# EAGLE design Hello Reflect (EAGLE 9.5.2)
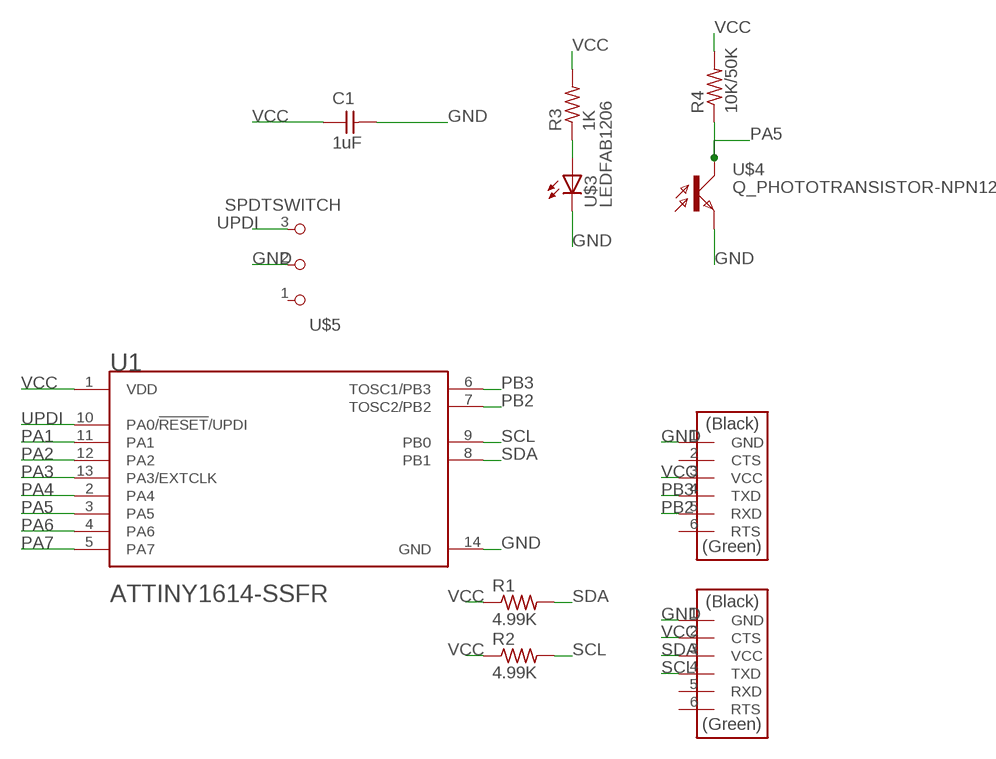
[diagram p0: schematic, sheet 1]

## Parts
C1  1uF  CAP_UNPOLARIZEDFAB  [C1206FAB]
R1  4.99K  R1206FAB  [R1206FAB]
R2  4.99K  R1206FAB  [R1206FAB]
R3  1K  R1206FAB  [R1206FAB]
R4  10K/50K  R1206FAB  [R1206FAB]
U1  MICROCHIP_ATTINY1614-SSFRMICROCHIP_ATTINY1614-SSFR_0_1  [MICROCHIP_ATTINY1614]
U$1  CONN_06_FTDI-SMD-HEADER  [1X06SMD]
U$2  CONN_06_FTDI-SMD-HEADER  [1X06SMD]
U$3  LEDFAB1206  [LED1206FAB]
U$4  Q_PHOTOTRANSISTOR-NPN1206  [OP1206]
U$5  SPDTSWITCH  [SPDTSWITCH]

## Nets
GND: C1.2 U1.14(GND) U$1.1(GND) U$2.1(GND) U$3.2(C) U$4.EMITTER(E) U$5.2
N$1: R3.1 U$3.1(A)
PA1: U1.11(PA1)
PA2: U1.12(PA2)
PA3: U1.13(PA3/EXTCLK)
PA4: U1.2(PA4)
PA5: R4.1 U1.3(PA5) U$4.COLLECTOR(C)
PA6: U1.4(PA6)
PA7: U1.5(PA7)
PB2: U1.7(TOSC2/PB2) U$2.5(RXD)
PB3: U1.6(TOSC1/PB3) U$2.4(TXD)
SCL: R2.2 U1.9(PB0) U$1.4(TXD)
SDA: R1.2 U1.8(PB1) U$1.3(VCC)
UPDI: U1.10(PA0/!RESET!/UPDI) U$5.3
VCC [New Class]: C1.1 R1.1 R2.1 R3.2 R4.2 U1.1(VDD) U$1.2(CTS) U$2.3(VCC)
Unconnected: U$1.5(RXD) U$1.6(RTS) U$2.2(CTS) U$2.6(RTS) U$5.1

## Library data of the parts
C1 = fab:CAP_UNPOLARIZED
R1-R4 = fab:R: Resistor (US Symbol)
U1 = Microchip - ATTINY1614-SSFR:MICROCHIP_ATTINY1614-SSFR: IC MCU 8BIT 16KB FLASH 14SOIC; AUTOMOTIVE: No; CENTROID_NOT_SPECIFIED: No; CORE_ARCHITECTURE: AVR; DATASHEET: http://ww1.microchip.com/downloads/en/DeviceDoc/ATtiny1614-DataSheet-DS40001995B.pdf; DATA_BUS_WIDTH: 8bits; DEVICE_CLASS_L1: Integrated Circuits (ICs); DEVICE_CLASS_L2: Embedded Processors and Controllers; DEVICE_CLASS_L3: Microcontrollers; DIGIKEY_DESCRIPTION: IC MCU 8BIT 16KB FLASH 14SOIC; DIGIKEY_PART_NUMBER: ATTINY1614-SSFRCT-ND; FOOTPRINT_PARAMETERS_1: {"fp_type":"SOIC_narrow","params":{"N":{"nom":14,"long name":"Number of leads","min":null,"max":null,"short name":"N","type":"count"},"A":{"nom":false,"long name":"Height","min":false,"max":1750000,"short name":"A","type":"measurement"},"A1":{"nom":false,"long name":"Package clearance","min":100000,"max":250000,"short name":"A1","type":"measurement"},"A2":{"nom":false,"long name":"Package height","min":1250000,"max":false,"short name":"A2","type":"measurement"},"D":{"nom":8650000,"long name":"Package length","min":8550000,"max":8750000,"short name":"D","type":"measurement"},"E":{"nom":6000000,"long name":"Width w/ leads","min":5800000,"max":6200000,"short name":"E","type":"measurement"},"E1":{"nom":3900000,"long name":"Package width","min":3800000,"max":4000000,"short name":"E1","type":"measurement"},"B":{"nom":false,"long name":"Lead width","min":310000,"max":510000,"short name":"B","type":"measurement"},"C":{"nom":false,"long name":"Lead thickness","min":100000,"max":250000,"short name":"C","type":"measurement"},"e":{"nom":1270000,"long name":"Lead pitch","min":null,"max":null,"short name":"e","type":"measurement"},"L":{"nom":false,"long name":"Lead foot length","min":400000,"max":1270000,"short name":"L","type":"measurement"},"PHI":{"nom":false,"long name":"Lead foot angle","min":0,"max":8000000,"short name":"PHI","type":"measurement"},"HT":{"default":"No","long name":"Thermal pad","type":"multichoiceparent","short name":"HT","children":[]},"offset x":{"nom":0,"long name":"X Center offset","min":null,"max":null,"short name":"offset x","type":"measurement"},"offset y":{"nom":0,"long name":"Y Center offset","min":null,"max":null,"short name":"offset y","type":"measurement"},"LS":{"default":"Rounded rectangle","long name":"Land shape","type":"multichoice","short name":"LS"},"LS1":{"default":"Rectangle","long name":"Land shape (Pin 1)","type":"multichoice","short name":"LS1"},"solder toe":{"nom":550000,"long name":"Solder fillet (toe)","min":null,"max":null,"short name":"solder toe","type":"fixedmeasurement"},"solder heel":{"nom":450000,"long name":"Solder fillet (heel)","min":null,"max":null,"short name":"solder heel","type":"fixedmeasurement"},"solder side":{"nom":50000,"long name":"Solder fillet (side)","min":null,"max":null,"short name":"solder side","type":"fixedmeasurement"},"courtyard":{"nom":500000,"long name":"Courtyard","min":null,"max":null,"short name":"courtyard","type":"fixedmeasurement"},"SF":{"default":"A","long name":"Packing level","type":"multichoiceparent","short name":"SF","help":"http://support.upverter.com/customer/portal/articles/978783-what-is-a-footprint-packing-level","children":["solder toe","solder heel","solder side","courtyard"]}}}; FOOTPRINT_PARAMETERS_2: {"fp_type":"SOIC_narrow","params":{"N":{"nom":14,"long name":"Number of leads","min":null,"max":null,"short name":"N","type":"count"},"A":{"nom":false,"long name":"Height","min":false,"max":1750000,"short name":"A","type":"measurement"},"A1":{"nom":false,"long name":"Package clearance","min":100000,"max":250000,"short name":"A1","type":"measurement"},"A2":{"nom":false,"long name":"Package height","min":1250000,"max":false,"short name":"A2","type":"measurement"},"D":{"nom":8650000,"long name":"Package length","min":8550000,"max":8750000,"short name":"D","type":"measurement"},"E":{"nom":6000000,"long name":"Width w/ leads","min":5800000,"max":6200000,"short name":"E","type":"measurement"},"E1":{"nom":3900000,"long name":"Package width","min":3800000,"max":4000000,"short name":"E1","type":"measurement"},"B":{"nom":false,"long name":"Lead width","min":310000,"max":510000,"short name":"B","type":"measurement"},"C":{"nom":false,"long name":"Lead thickness","min":100000,"max":250000,"short name":"C","type":"measurement"},"e":{"nom":1270000,"long name":"Lead pitch","min":null,"max":null,"short name":"e","type":"measurement"},"L":{"nom":false,"long name":"Lead foot length","min":400000,"max":1270000,"short name":"L","type":"measurement"},"PHI":{"nom":false,"long name":"Lead foot angle","min":0,"max":8000000,"short name":"PHI","type":"measurement"},"HT":{"default":"No","long name":"Thermal pad","type":"multichoiceparent","short name":"HT","children":[]},"offset x":{"nom":0,"long name":"X Center offset","min":null,"max":null,"short name":"offset x","type":"measurement"},"offset y":{"nom":0,"long name":"Y Center offset","min":null,"max":null,"short name":"offset y","type":"measurement"},"LS":{"default":"Rounded rectangle","long name":"Land shape","type":"multichoice","short name":"LS"},"LS1":{"default":"Rectangle","long name":"Land shape (Pin 1)","type":"multichoice","short name":"LS1"},"solder toe":{"nom":350000,"long name":"Solder fillet (toe)","min":null,"max":null,"short name":"solder toe","type":"fixedmeasurement"},"solder heel":{"nom":350000,"long name":"Solder fillet (heel)","min":null,"max":null,"short name":"solder heel","type":"fixedmeasurement"},"solder side":{"nom":30000,"long name":"Solder fillet (side)","min":null,"max":null,"short name":"solder side","type":"fixedmeasurement"},"courtyard":{"nom":250000,"long name":"Courtyard","min":null,"max":null,"short name":"courtyard","type":"fixedmeasurement"},"SF":{"default":"B","long name":"Packing level","type":"multichoiceparent","short name":"SF","help":"http://support.upverter.com/customer/portal/articles/978783-what-is-a-footprint-packing-level","children":["solder toe","solder heel","solder side","courtyard"]}}}; FOOTPRINT_PARAMETERS_3: {"fp_type":"SOIC_narrow","params":{"N":{"nom":14,"long name":"Number of leads","min":null,"max":null,"short name":"N","type":"count"},"A":{"nom":false,"long name":"Height","min":false,"max":1750000,"short name":"A","type":"measurement"},"A1":{"nom":false,"long name":"Package clearance","min":100000,"max":250000,"short name":"A1","type":"measurement"},"A2":{"nom":false,"long name":"Package height","min":1250000,"max":false,"short name":"A2","type":"measurement"},"D":{"nom":8650000,"long name":"Package length","min":8550000,"max":8750000,"short name":"D","type":"measurement"},"E":{"nom":6000000,"long name":"Width w/ leads","min":5800000,"max":6200000,"short name":"E","type":"measurement"},"E1":{"nom":3900000,"long name":"Package width","min":3800000,"max":4000000,"short name":"E1","type":"measurement"},"B":{"nom":false,"long name":"Lead width","min":310000,"max":510000,"short name":"B","type":"measurement"},"C":{"nom":false,"long name":"Lead thickness","min":100000,"max":250000,"short name":"C","type":"measurement"},"e":{"nom":1270000,"long name":"Lead pitch","min":null,"max":null,"short name":"e","type":"measurement"},"L":{"nom":false,"long name":"Lead foot length","min":400000,"max":1270000,"short name":"L","type":"measurement"},"PHI":{"nom":false,"long name":"Lead foot angle","min":0,"max":8000000,"short name":"PHI","type":"measurement"},"HT":{"default":"No","long name":"Thermal pad","type":"multichoiceparent","short name":"HT","children":[]},"offset x":{"nom":0,"long name":"X Center offset","min":null,"max":null,"short name":"offset x","type":"measurement"},"offset y":{"nom":0,"long name":"Y Center offset","min":null,"max":null,"short name":"offset y","type":"measurement"},"LS":{"default":"Rounded rectangle","long name":"Land shape","type":"multichoice","short name":"LS"},"LS1":{"default":"Rectangle","long name":"Land shape (Pin 1)","type":"multichoice","short name":"LS1"},"solder toe":{"nom":150000,"long name":"Solder fillet (toe)","min":null,"max":null,"short name":"solder toe","type":"fixedmeasurement"},"solder heel":{"nom":250000,"long name":"Solder fillet (heel)","min":null,"max":null,"short name":"solder heel","type":"fixedmeasurement"},"solder side":{"nom":10000,"long name":"Solder fillet (side)","min":null,"max":null,"short name":"solder side","type":"fixedmeasurement"},"courtyard":{"nom":100000,"long name":"Courtyard","min":null,"max":null,"short name":"courtyard","type":"fixedmeasurement"},"SF":{"default":"C","long name":"Packing level","type":"multichoiceparent","short name":"SF","help":"http://support.upverter.com/customer/portal/articles/978783-what-is-a-footprint-packing-level","children":["solder toe","solder heel","solder side","courtyard"]}}}; FOOTPRINT_VARIANT_NAME_0: Recommended_Land_Pattern; FOOTPRINT_VARIANT_NAME_1: IPC_A; FOOTPRINT_VARIANT_NAME_2: IPC_B; FOOTPRINT_VARIANT_NAME_3: IPC_C; FREQUENCY: 16MHz; HEIGHT: 1.75mm; INTERFACE: I2C,SPI,UART,USART,2-Wire,LIN,IrDA; IPC_LAND_PATTERN_NAME: SOIC127P600X175-14; LEAD_FREE: Yes; MAX_SUPPLY_VOLTAGE: 5.5V; MEMORY_SIZE: 16KBytes; MEMORY_TYPE: FLASH; MF: Microchip; MFG_PACKAGE_IDENT: C04-065-D3X; MFG_PACKAGE_IDENT_DATE: 0; MFG_PACKAGE_IDENT_REV: D; MIN_SUPPLY_VOLTAGE: 1.8V; MOUSER_DESCRIPTION: 8-Bit AVR Microcontroller 16Kbyte Flash 2Kbyte SRAM 14-Pin SOIC T/R; MOUSER_PART_NUMBER: 556-ATTINY1614SSFR; MPN: ATTINY1614-SSFR; NOMINAL_SUPPLY_CURRENT: 2.6-10200uA; NUMBER_OF_A/D_CONVERTERS: 2; NUMBER_OF_ADC_CHANNELS: 14; NUMBER_OF_CORES: 1; NUMBER_OF_I/OS: 12; NUMBER_OF_I2C_CHANNELS: 1; NUMBER_OF_PWM_CHANNELS: 1; NUMBER_OF_SPI_CHANNELS: 1; NUMBER_OF_TIMERS/COUNTERS: 5; NUMBER_OF_UART_CHANNELS: 1; PACKAGE: SOIC14; PREFIX: U; RAM_SIZE: 2KBytes; ROHS: Yes; STANDOFF_HEIGHT: 0.1mm; TEMPERATURE_RANGE_HIGH: +125°C; TEMPERATURE_RANGE_LOW: -40°C; VERIFICATION_VERSION: 0.0.0.3
U$1 U$2 = fab:CONN_06_FTDI-SMD-HEADER
U$3 = fab:LED: LED
U$4 = fab:Q_PHOTOTRANSISTOR-NPN
U$5 = fab:SPDTSWITCH

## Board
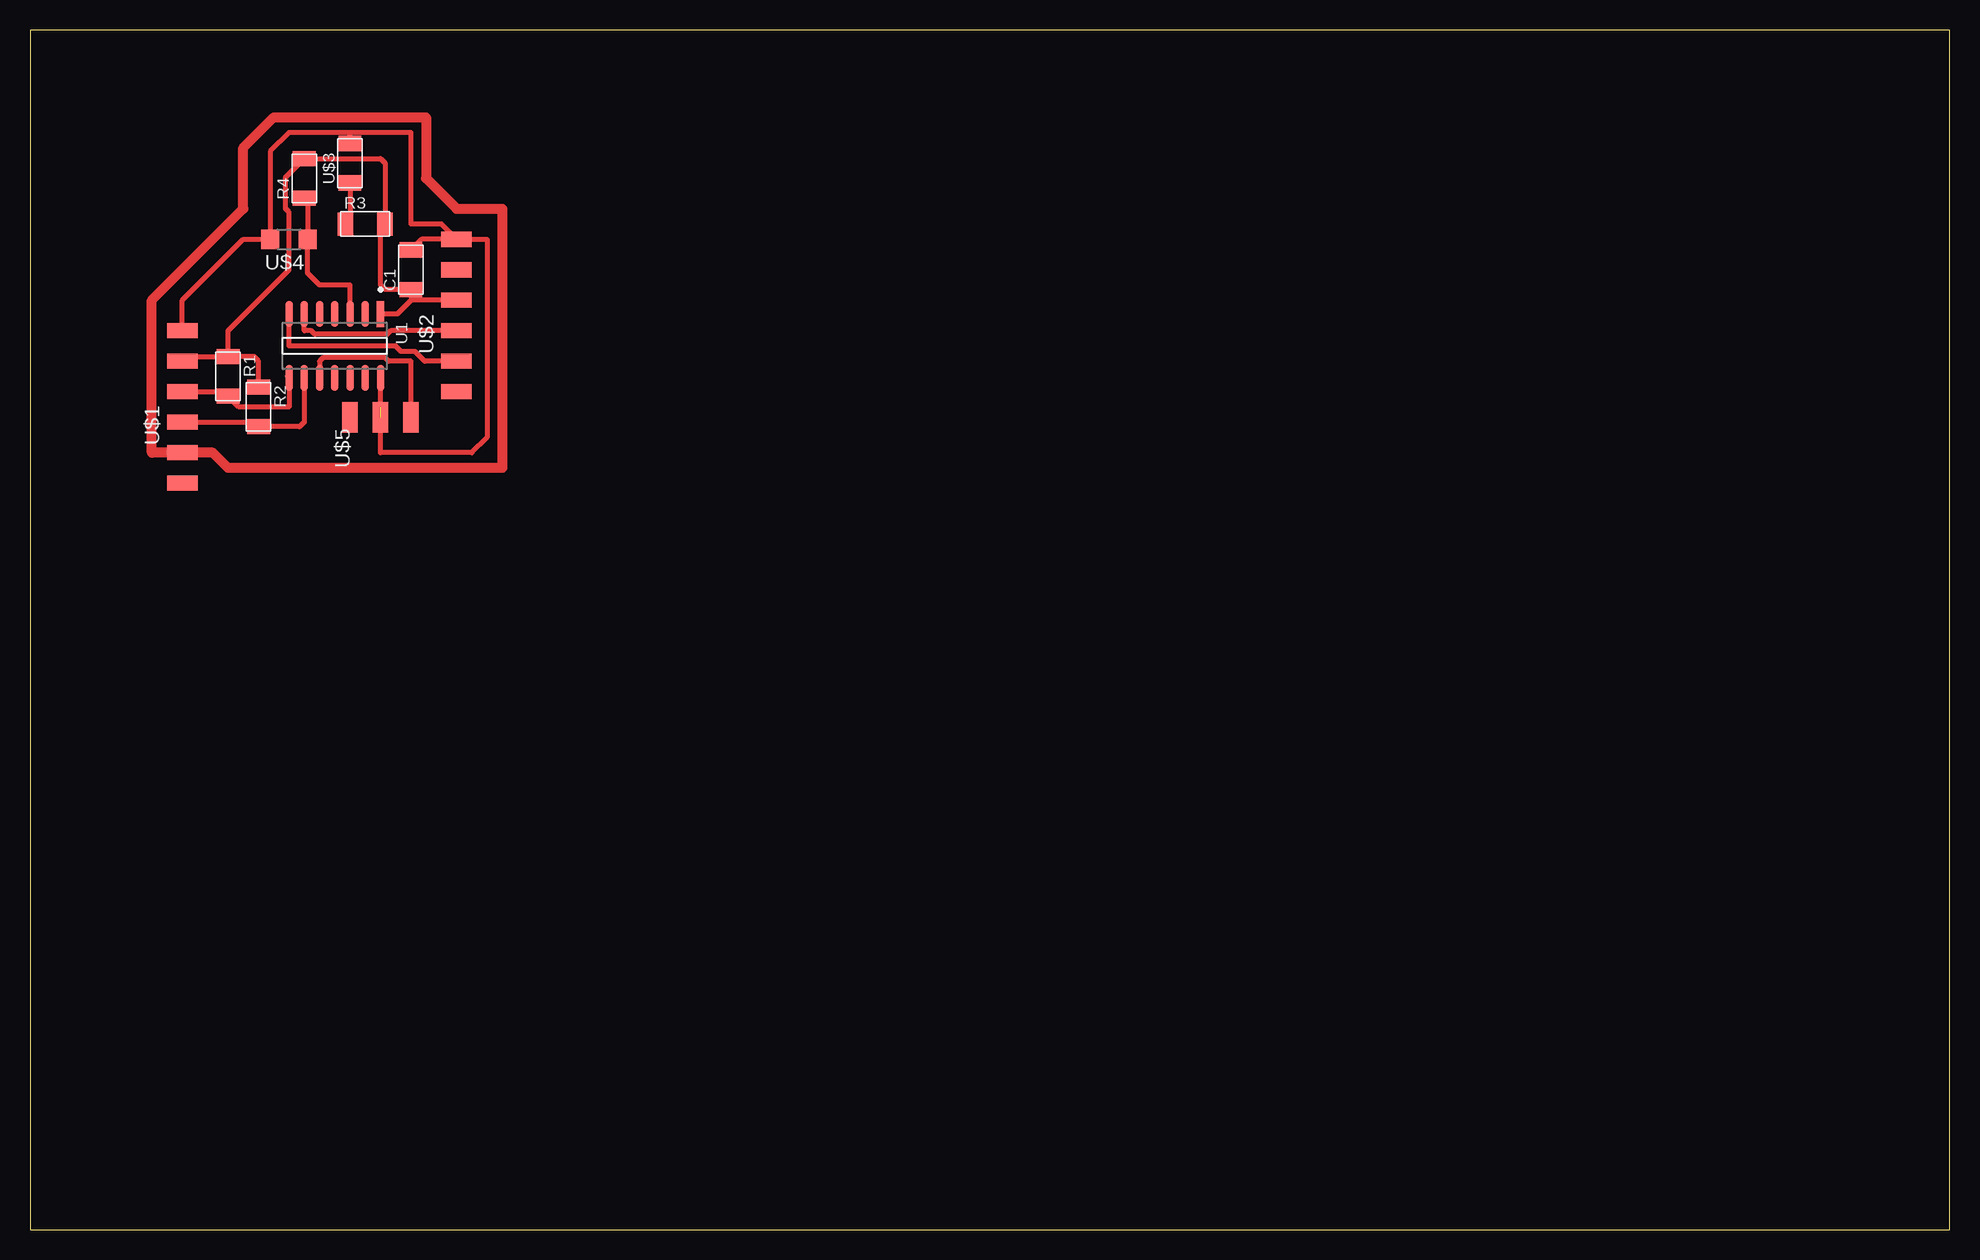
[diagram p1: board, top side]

Size 160 x 100 mm. Coordinates in mm from the lower left corner, seen from the top.
Outline: 0,0 160,0 160,100 0,100 0,0
Copper layers (1*16): Top 0.035mm / dielectric 1.5mm / Bottom 0.035mm
Design rules "default *": minimum track width 16mil, minimum drill 0.35mm, track to track 16mil, track to pad 16mil, pad to pad 16mil, via to via 16mil, smd to smd 16mil, copper to edge 40mil, drill to drill 6mil, minimum pad ring 10mil, minimum via ring 8mil, stop-mask expansion 4mil, vias tented up to drill 0mil, thermal gap 10mil

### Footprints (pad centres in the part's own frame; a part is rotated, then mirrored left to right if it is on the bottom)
C1206FAB = smd 1.27 x 1.905: 1 -1.651,0; 2 1.651,0
R1206FAB = smd 1.27 x 1.905: 1 -1.651,0; 2 1.651,0
MICROCHIP_ATTINY1614 = smd 2.169 x 0.622: 1 -2.67,3.81; 2 -2.67,2.54; 3 -2.67,1.27; 4 -2.67,0; 5 -2.67,-1.27; 6 -2.67,-2.54; 7 -2.67,-3.81; 8 2.67,-3.81; 9 2.67,-2.54; 10 2.67,-1.27; 11 2.67,0; 12 2.67,1.27; 13 2.67,2.54; 14 2.67,3.81
1X06SMD = smd 2.54 x 1.27: 1 0,6.35; 2 0,3.81; 3 0,1.27; 4 0,-1.27; 5 0,-3.81; 6 0,-6.35
LED1206FAB = smd 1.27 x 1.905: 1 -1.651,0; 2 1.651,0
OP1206 = smd 1.5 x 1.6: COLLECTOR -1.55,0; EMITTER 1.55,0
SPDTSWITCH = smd 2.54 x 1.27: 1 0.38,2.54; 2 0.38,0; 3 0.38,-2.54

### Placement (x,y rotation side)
C1  31.75,80.01 90 top
R1  16.51,71.12 270 top
R2  19.05,68.58 270 top
R3  27.94,83.82 0 top
R4  22.86,87.63 90 top
U1  25.4,73.66 270 top
U$1  12.7,68.58 0 top
U$2  35.56,76.2 0 top
U$3  26.67,88.9 90 top
U$4  21.59,82.55 180 top
U$5  29.21,67.31 90 top

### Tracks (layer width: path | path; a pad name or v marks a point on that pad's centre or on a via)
GND  (1 unrouted)
  Top 0.406: U$2.1 32.64,82.55 C1.2 | U$2.1 38.1,82.55 38.1,66.04 36.83,64.77 29.21,64.77 U$5.2 | 29.21,68.58 U1.14 | U$1.1 12.7,77.47 17.78,82.55 U$4.EMITTER 20.04,89.89 21.59,91.44 26.67,91.44 | U$2.1 34.29,83.82 31.75,83.82 31.75,91.44 26.67,91.44 | U$3.2 26.67,91.44
N$1
  Top 0.406: U$3.1 26.67,84.2 R3.1
N$2
  Top 0.813: 17.78,85.09 17.78,90.17 20.32,92.71 33.02,92.71 33.02,87.63 35.56,85.09 39.37,85.09 39.37,63.5 16.51,63.5 15.24,64.77 10.16,64.77 10.16,77.47 17.78,85.09
PA5
  Top 0.406: U1.3 26.67,78.74 24.13,78.74 23.14,79.73 U$4.COLLECTOR 23.14,85.7 R4.1
PB2
  Top 0.406: U$2.5 32.9,72.39 32.09,73.2 30.94,73.2 30.48,73.66 21.59,73.66 U1.7
PB3
  Top 0.406: U$2.4 30.07,74.93 29.77,74.64 23.75,74.64 23.45,74.93 22.86,74.93 U1.6
SCL
  Top 0.406: U1.9 22.86,67.31 22.48,66.93 R2.2 18.67,67.31 U$1.4
SDA
  Top 0.406: 21.46,71.12 U1.8 21.59,68.58 17.4,68.58 R1.2 16.13,69.85 U$1.3
UPDI
  Top 0.406: U$5.3 31.75,72.39 29.89,72.39 29.59,72.68 24.42,72.68 24.13,72.39 U1.10
VCC
  Top 0.406: U$2.3 31.75,77.47 | 31.75,77.47 C1.1 29.59,78.36 29.21,78.74 29.21,83.44 R3.2 29.59,88.9 29.21,89.28 R4.2 | 31.75,77.47 30.61,76.33 U1.1 | R2.1 19.05,72.39 18.67,72.77 R1.1 | U$1.2 13.08,72.77 R1.1 | R4.2 22.48,88.9 | R1.1 16.51,74.93 21.59,80.01 21.59,84.8 21.3,85.09 21.3,87.72 R4.2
